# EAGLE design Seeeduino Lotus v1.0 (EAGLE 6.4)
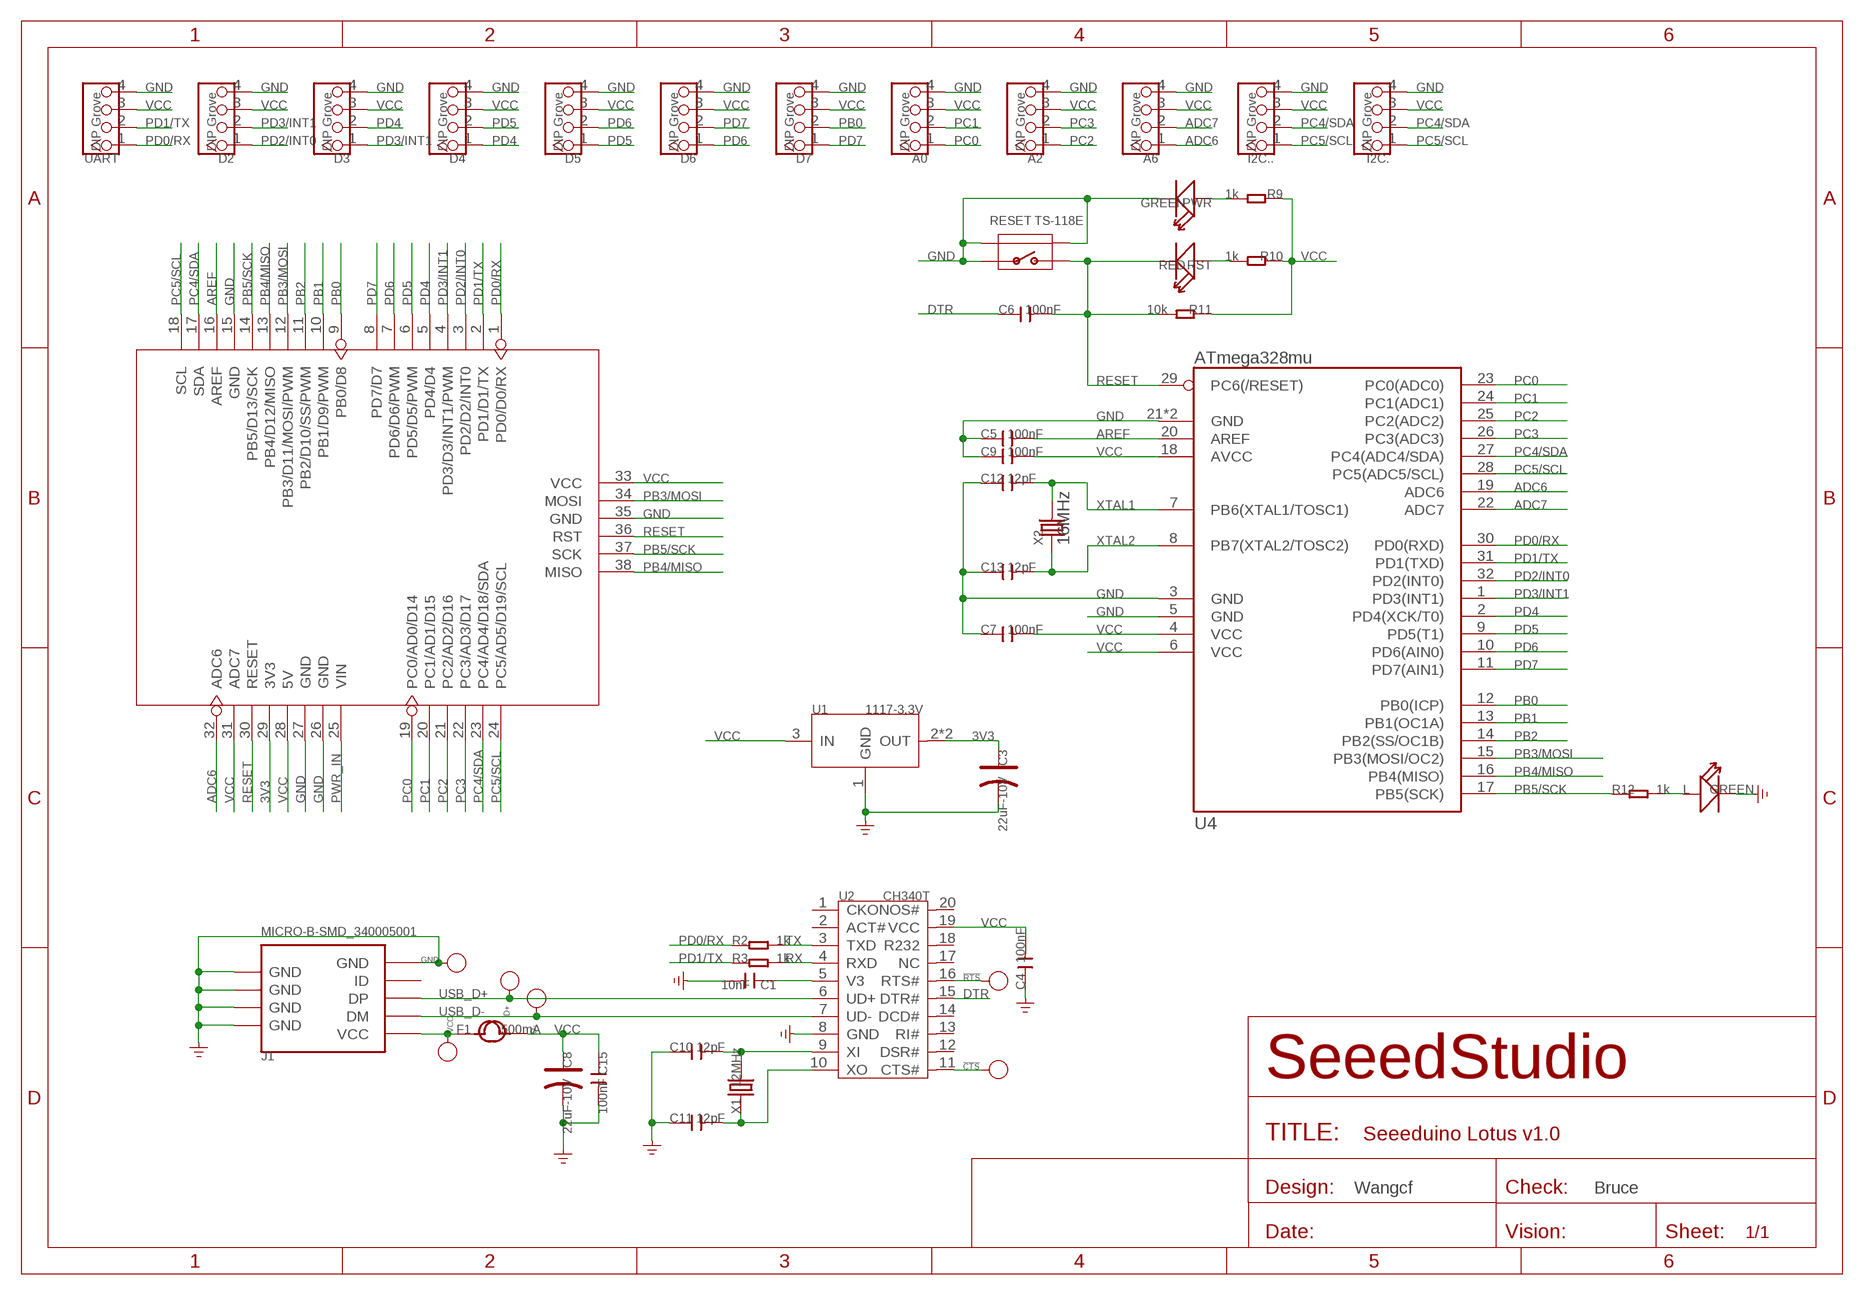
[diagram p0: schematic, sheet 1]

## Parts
!CTS  PAD-TEST-POINT'4545'  [TP_4545]
!RTS  PAD-TEST-POINT'4545'  [TP_4545]
A0  DIP Grove  TWIG-4P-2.0-2.0  [4P-2.0]
A2  DIP Grove  TWIG-4P-2.0-2.0  [4P-2.0]
A6  DIP Grove  TWIG-4P-2.0-2.0  [4P-2.0]
C1  10nF  C-0603  [C0603]
C3  22uF-10V  CAP-AVX-A  [AVX-A]
C4  100nF  C-0603  [C0603]
C5  100nF  C-0603  [C0603]
C6  100nF  C-0603  [C0603]
C7  100nF  C-0603  [C0603]
C8  22uF-10V  CAP-AVX-A  [AVX-A]
C9  100nF  C-0603  [C0603]
C10  12pF  C-0603  [C0603]
C11  12pF  C-0603  [C0603]
C12  12pF  C-0603  [C0603]
C13  12pF  C-0603  [C0603]
C15  100nF  C-0603  [C0603]
D2  DIP Grove  TWIG-4P-2.0-2.0  [4P-2.0]
D3  DIP Grove  TWIG-4P-2.0-2.0  [4P-2.0]
D4  DIP Grove  TWIG-4P-2.0-2.0  [4P-2.0]
D5  DIP Grove  TWIG-4P-2.0-2.0  [4P-2.0]
D6  DIP Grove  TWIG-4P-2.0-2.0  [4P-2.0]
D7  DIP Grove  TWIG-4P-2.0-2.0  [4P-2.0]
D+  PAD-TEST-POINT'4545'  [TP_4545]
D-  PAD-TEST-POINT'4545'  [TP_4545]
F1  500mA  FUSE'1206'  [F1206]
GND  PAD-TEST-POINT'4545'  [TP_4545]
I2C.  DIP Grove  TWIG-4P-2.0-2.0  [4P-2.0]
I2C..  DIP Grove  TWIG-4P-2.0-2.0  [4P-2.0]
J1  MICRO-B-SMD_340005001  USB-MINIUSB-5P-MICRO  [MICRO-USB]
L  GREEN  LED'0603'  [LED-0603]
PWR  GREEN  LED'0603'  [LED-0603]
R2  1k  R-0603  [R0603]
R3  1k  R-0603  [R0603]
R9  1k  R-0603  [R0603]
R10  1k  R-0603  [R0603]
R11  10k  R-0603  [R0603]
R12  1k  R-0603  [R0603]
RESET  TS-118E  BUTTON-4P-REINFORCE'TS-1188E'  [4P-SMD-7X3.5X3.5H]
RST  RED  LED'0603'  [LED-0603]
U1  1117-3.3V  LD1117'SOT89'  [SOT89]
U2  CH340T  [SSOP20]
U3  ARDUINO-38P  [ARDUINO-38P]
U4  ATmega328mu  ATMEGA8/168/328MLF  [MLF32X-W/HEAT]
UART  DIP Grove  TWIG-4P-2.0-2.0  [4P-2.0]
VCC  PAD-TEST-POINT'4545'  [TP_4545]
X1  12MHz  CRYSTAL'5032'  [2P-SMD-5X3.2]
X2  16MHz  CRYSTAL'5032'  [2P-SMD-5X3.2]

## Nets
3V3: C3.+ U1.2(OUT) U1.4(OUT) U3.29(3V3)
ADC6: A6.1 U3.32(ADC6) U4.19(ADC6)
ADC7: A6.2 U4.22(ADC7)
AREF: C5.2 U3.16(AREF) U4.20(AREF)
CTS: !CTS.T U2.11(CTS#)
DTR: C6.1 U2.15(DTR#)
GND: A0.4 A2.4 A6.4 C1.2 C3.- C4.1 C5.1 C7.1 C8.- C9.1 C10.1 C11.1 C12.1 C13.1 C15.2 D2.4 D3.4 D4.4 D5.4 D6.4 D7.4 GND.T I2C..4 I2C...4 J1.5(GND) J1.S1(GND) J1.S2(GND) J1.S3(GND) J1.S4(GND) J1.S5(GND) J1.S6(GND) L.- PWR.- RESET.1 RESET.S1 RESET.S2 U1.1(GND) U2.8(GND) U3.15(GND) U3.26(GND) U3.27(GND) U3.35(GND) U4.3(GND) U4.5(GND) U4.21(GND) U4.HEAT(GND) UART.4
N$2: R10.2 RST.+
N$3: PWR.+ R9.2
N$4: C10.2 U2.9(XI) X1.2
N$5: C11.2 U2.10(XO) X1.1
N$11: !RTS.T U2.16(RTS#)
N$12 [usbvcc]: F1.1 J1.1(VCC) VCC.T
N$13: L.+ R12.2
PB0: D7.2 U3.9(PB0/D8) U4.12(PB0(ICP))
PB1: U3.10(PB1/D9/PWM) U4.13(PB1(OC1A))
PB2: U3.11(PB2/D10/SS/PWM) U4.14(PB2(SS/OC1B))
PB3/MOSI: U3.12(PB3/D11/MOSI/PWM) U3.34(MOSI) U4.15(PB3(MOSI/OC2))
PB4/MISO: U3.13(PB4/D12/MISO) U3.38(MISO) U4.16(PB4(MISO))
PB5/SCK: R12.1 U3.14(PB5/D13/SCK) U3.37(SCK) U4.17(PB5(SCK))
PC0: A0.1 U3.19(PC0/AD0/D14) U4.23(PC0(ADC0))
PC1: A0.2 U3.20(PC1/AD1/D15) U4.24(PC1(ADC1))
PC2: A2.1 U3.21(PC2/AD2/D16) U4.25(PC2(ADC2))
PC3: A2.2 U3.22(PC3/AD3/D17) U4.26(PC3(ADC3))
PC4/SDA: I2C..2 I2C...2 U3.17(SDA) U3.23(PC4/AD4/D18/SDA) U4.27(PC4(ADC4/SDA))
PC5/SCL: I2C..1 I2C...1 U3.18(SCL) U3.24(PC5/AD5/D19/SCL) U4.28(PC5(ADC5/SCL))
PD0/RX: R2.1 U3.1(PD0/D0/RX) U4.30(PD0(RXD)) UART.1
PD1/TX: R3.1 U3.2(PD1/D1/TX) U4.31(PD1(TXD)) UART.2
PD2/INT0: D2.1 U3.3(PD2/D2/INT0) U4.32(PD2(INT0))
PD3/INT1: D2.2 D3.1 U3.4(PD3/D3/INT1/PWM) U4.1(PD3(INT1))
PD4: D3.2 D4.1 U3.5(PD4/D4) U4.2(PD4(XCK/T0))
PD5: D4.2 D5.1 U3.6(PD5/D5/PWM) U4.9(PD5(T1))
PD6: D5.2 D6.1 U3.7(PD6/D6/PWM) U4.10(PD6(AIN0))
PD7: D6.2 D7.1 U3.8(PD7/D7) U4.11(PD7(AIN1))
PWR_IN: U3.25(VIN)
RESET: C6.2 R11.2 RESET.2 RST.- U3.30(RESET) U3.36(RST) U4.29(PC6(/RESET))
RX: R3.2 U2.4(RXD)
TX: R2.2 U2.3(TXD)
USB_D+: D+.T J1.3(DP) U2.6(UD+)
USB_D-: D-.T J1.2(DM) U2.7(UD-)
V3: C1.1 U2.5(V3)
VCC: A0.3 A2.3 A6.3 C4.2 C7.2 C8.+ C9.2 C15.1 D2.3 D3.3 D4.3 D5.3 D6.3 D7.3 F1.2 I2C..3 I2C...3 R9.1 R10.1 R11.1 U1.3(IN) U2.19(VCC) U3.28(5V) U3.31(ADC7) U3.33(VCC) U4.4(VCC) U4.6(VCC) U4.18(AVCC) UART.3
XTAL1: C12.2 U4.7(PB6(XTAL1/TOSC1)) X2.2
XTAL2: C13.2 U4.8(PB7(XTAL2/TOSC2)) X2.1
Unconnected: J1.4(ID) U2.1(CKO) U2.2(ACT#) U2.12(DSR#) U2.13(RI#) U2.14(DCD#) U2.17(NC) U2.18(R232) U2.20(NOS#)

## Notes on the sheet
- Wangcf | Bruce

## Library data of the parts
!CTS !RTS D+ D- GND VCC = Discrete:PAD-TEST-POINT; PARTNO: DNP
A0 A2 A6 = Connector :TWIG-4P-2.0
C1 C4-C7 C9-C13 C15 = Discrete:C*: Ceramic Capacitors
C3 C8 = Discrete:CAP*: Electrolytic Capacitors,Tantalum Capacitors and Super Capacitors
D2-D7 I2C. I2C.. UART = Connector:TWIG-4P-2.0
F1 = Discrete:FUSE
J1 = Connector :USB-MINIUSB-5P
L PWR RST = Discrete:LED*
R2 R3 R9-R12 = Discrete:R*
RESET = Discrete:BUTTON-4P-REINFORCE: TS-1188E http://www.best-dz.com/?thread-374-2.html
U1 = IC:LD1117: Low Drop Fixed And Adjustable Positive Voltage Regulators http://www.datasheetcatalog.org/datasheet/SGSThomsonMicroelectronics/mXuqtqv.pdf
U2 = template:CH340T
U3 = moudle:ARDUINO-38P
U4 = IC:ATMEGA8/168/328: MICROCONTROLLER
X1 X2 = Discrete:CRYSTAL*: CRYSTAL

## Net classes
0 default: width 0.152 mm, drill 0.305 mm, clearance 0.152 mm
3 usbvcc: width 0.203 mm, drill 0.305 mm, clearance 0.203 mm

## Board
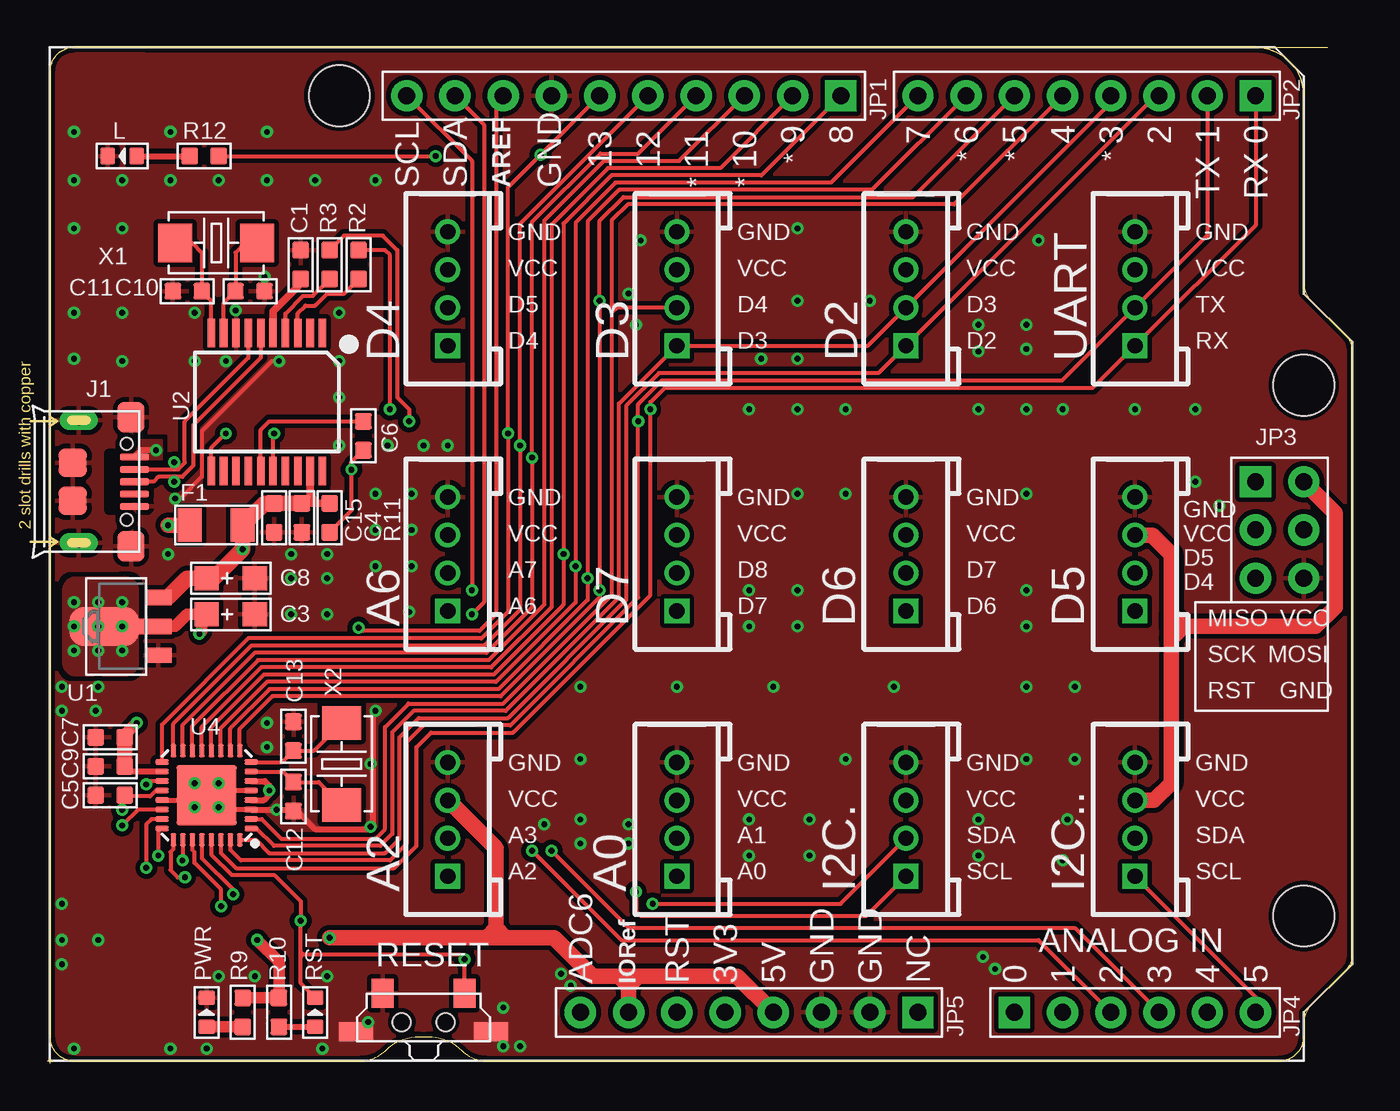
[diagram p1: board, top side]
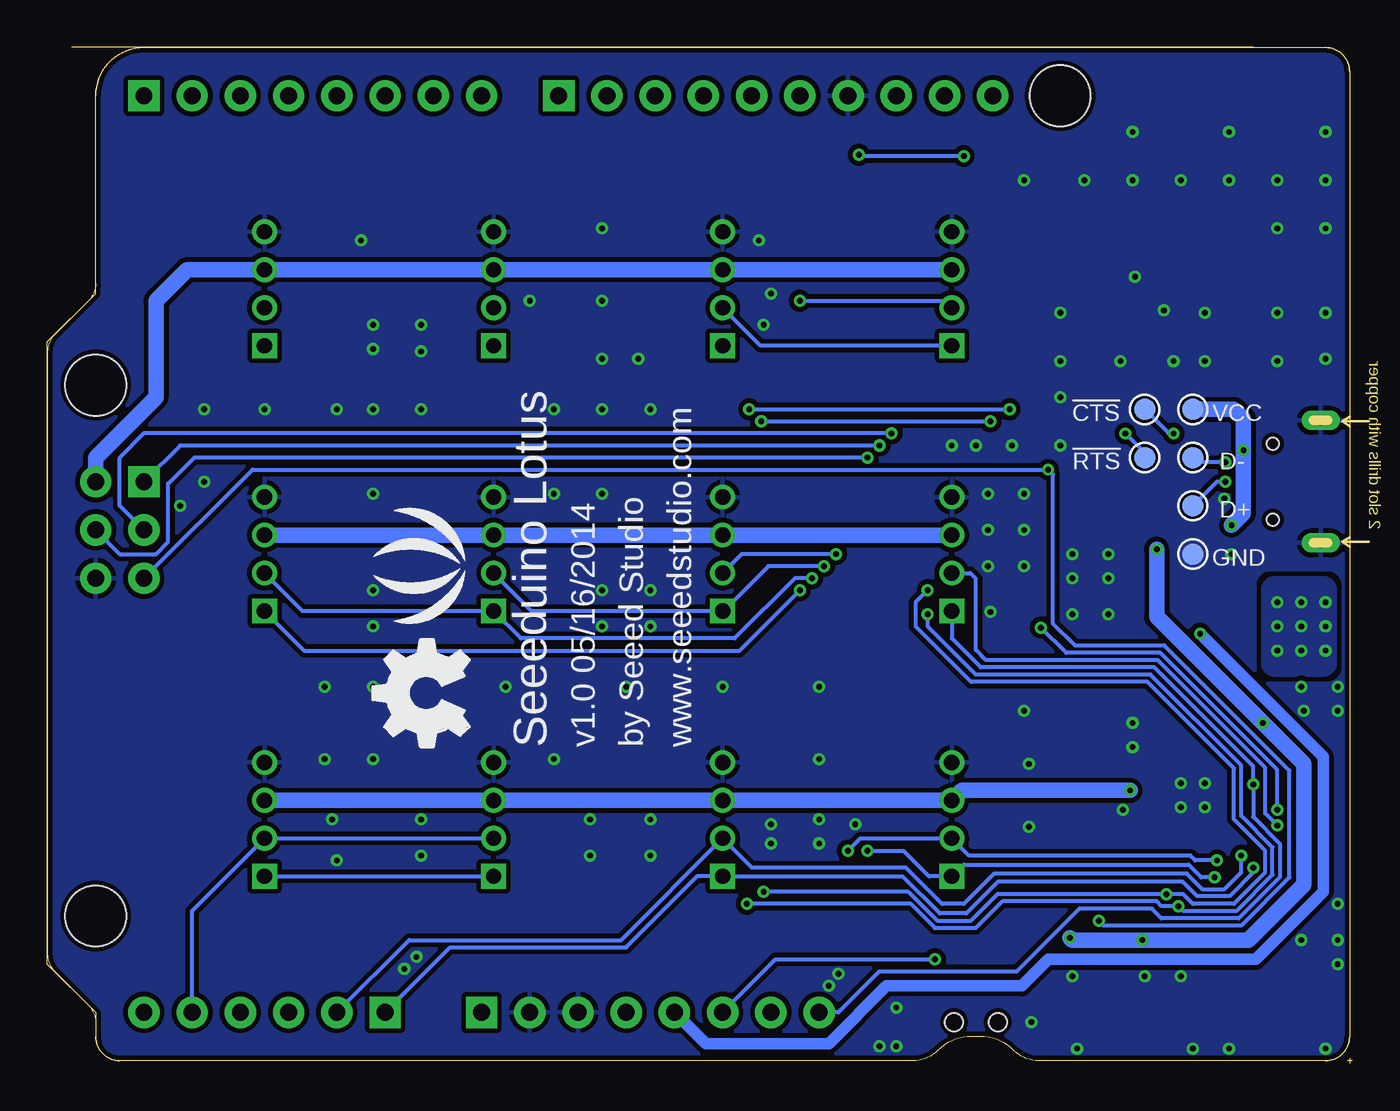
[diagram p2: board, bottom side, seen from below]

Size 68.71 x 53.47 mm. Coordinates in mm from the lower left corner, seen from the top.
Outline: 54 segments
Copper layers (1*16): Top 0.035mm / dielectric 1.5mm / Bottom 0.035mm
Design rules "SeeedStudio_rule_no_angle_090911 *": minimum track width 6mil, minimum drill 12mil, track to track 6mil, track to pad 6mil, pad to pad 6mil, via to via 6mil, smd to smd 0mil, copper to edge 10mil, drill to drill 10mil, minimum pad ring 10mil, minimum via ring 6mil, stop-mask expansion 2mil, vias tented up to drill 100mil, thermal gap 10mil

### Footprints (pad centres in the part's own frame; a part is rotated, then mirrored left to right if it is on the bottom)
TP_4545 = smd 1.143 x 1.143: T 0,0
4P-2.0 = drill 0.8 pad 1.27 square: 1 -3,0 | drill 0.8 pad 1.27: 2 -1,0; 3 1,0; 4 3,0
C0603 = smd 0.889 x 0.889: 1 -0.762,0; 2 0.762,0
AVX-A = smd 1.27 x 1.27: + -1.27,0; - 1.27,0
F1206 = smd 1.27 x 1.778: 1 -1.397,0; 2 1.397,0
MICRO-USB = smd 0.381 x 1.524: 1 -1.3,-0.25; 2 -0.65,-0.25; 3 0,-0.25; 4 0.65,-0.25; 5 1.3,-0.25 | smd 1.6 x 1.397: S1 -3.4,-0.427; S6 3.4,-0.427 | drill 0.508 pad 1.016 long: S2 -3.226,-3.175; S5 3.226,-3.175 | smd 1.5 x 1.5: S3 -1,-3.5; S4 1,-3.5 | hole 0.635: -2,-0.65; 2,-0.65
LED-0603 = smd 0.762 x 0.889: + -0.762,0; - 0.762,0
R0603 = smd 0.889 x 0.889: 1 -0.762,0; 2 0.762,0
4P-SMD-7X3.5X3.5H = smd 1.143 x 1.524: 1 -2.159,1.524; 2 2.159,1.524 | smd 1.778 x 1.016: S1 -3.556,-0.508; S2 3.556,-0.508 | hole 0.95: -1.15,0; 1.15,0
SOT89 = smd 0.8 x 1.4: 1 -1.524,-1.905; 3 1.524,-1.905 | smd 0.8 x 1.9: 2 0,-1.651 | smd 2.032 x 3.65: 4 0,0.94
SSOP20 = smd 0.4 x 1.5: 1 -2.925,-3.625; 2 -2.275,-3.625; 3 -1.625,-3.625; 4 -0.975,-3.625; 5 -0.325,-3.625; 6 0.325,-3.625; 7 0.975,-3.625; 8 1.625,-3.625; 9 2.275,-3.625; 10 2.925,-3.625; 11 2.925,3.625; 12 2.275,3.625; 13 1.625,3.625; 14 0.975,3.625; 15 0.325,3.625; 16 -0.325,3.625; 17 -0.975,3.625; 18 -1.625,3.625; 19 -2.275,3.625; 20 -2.925,3.625
ARDUINO-38P = drill 0.889 pad 1.651 square: 1 63.5,50.8; 9 41.656,50.8; 19 50.8,2.54; 25 45.72,2.54; 38 63.5,30.48 | drill 0.889 pad 1.651: 2 60.96,50.8; 3 58.42,50.8; 4 55.88,50.8; 5 53.34,50.8; 6 50.8,50.8; 7 48.26,50.8; 8 45.72,50.8; 10 39.116,50.8; 11 36.576,50.8; 12 34.036,50.8; 13 31.496,50.8; 14 28.956,50.8; 15 26.416,50.8; 16 23.876,50.8; 17 21.336,50.8; 18 18.796,50.8; 20 53.34,2.54; 21 55.88,2.54; 22 58.42,2.54; 23 60.96,2.54; 24 63.5,2.54; 26 43.18,2.54; 27 40.64,2.54; 28 38.1,2.54; 29 35.56,2.54; 30 33.02,2.54; 31 30.48,2.54; 32 27.94,2.54; 33 66.04,30.48; 34 66.04,27.94; 35 66.04,25.4; 36 63.5,25.4; 37 63.5,27.94 | hole 3.2: 15.24,50.8; 66.04,35.56; 66.04,7.62
MLF32X-W/HEAT = smd 0.7 x 0.3: 1 -2.35,1.75; 2 -2.35,1.25; 3 -2.35,0.75; 4 -2.35,0.25; 5 -2.35,-0.25; 6 -2.35,-0.75; 7 -2.35,-1.25; 8 -2.35,-1.75; 17 2.35,-1.75; 18 2.35,-1.25; 19 2.35,-0.75; 20 2.35,-0.25; 21 2.35,0.25; 22 2.35,0.75; 23 2.35,1.25; 24 2.35,1.75 | smd 0.3 x 0.7: 9 -1.75,-2.35; 10 -1.25,-2.35; 11 -0.75,-2.35; 12 -0.25,-2.35; 13 0.25,-2.35; 14 0.75,-2.35; 15 1.25,-2.35; 16 1.75,-2.35; 25 1.75,2.35; 26 1.25,2.35; 27 0.75,2.35; 28 0.25,2.35; 29 -0.25,2.35; 30 -0.75,2.35; 31 -1.25,2.35; 32 -1.75,2.35 | smd 3.175 x 3.175: HEAT 0,0
2P-SMD-5X3.2 = smd 1.778 x 2.032: 1 -2.159,0; 2 2.159,0

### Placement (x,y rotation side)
!CTS  10.92,34.42 0 bottom
!RTS  10.92,31.88 0 bottom
A0  33.15,12.83 90 top
A2  21.08,12.83 90 top
A6  21.08,26.8 90 top
C1  13.34,42.04 90 top
C3  9.65,23.62 0 top
C4  13.4,28.7 90 top
C5  3.3,14.1 0 top
C6  16.64,33.02 270 top
C7  3.3,17.14 0 top
C8  9.65,25.53 0 top
C9  3.3,15.62 0 top
C10  10.67,40.64 180 top
C11  7.37,40.64 0 top
C12  12.95,14.03 90 top
C13  12.95,17.21 270 top
C15  11.94,28.7 270 top
D2  45.21,40.77 90 top
D3  33.15,40.77 90 top
D4  21.08,40.77 90 top
D5  57.28,26.8 90 top
D6  45.21,26.8 90 top
D7  33.15,26.8 90 top
D+  8.38,29.34 0 bottom
D-  8.38,31.88 0 bottom
F1  8.89,28.32 0 top
GND  8.38,26.8 0 bottom
I2C.  45.21,12.83 90 top
I2C..  57.28,12.83 90 top
J1  4.83,30.61 270 top
L  3.94,47.75 180 top
PWR  8.38,2.67 90 top
R2  16.38,42.04 270 top
R3  14.86,42.04 270 top
R9  10.29,2.67 270 top
R10  12.19,2.67 270 top
R11  14.86,28.7 270 top
R12  8.26,47.75 180 top
RESET  19.81,2.16 0 top
RST  14.1,2.67 90 top
U1  3.94,22.99 90 top
U2  11.56,34.8 180 top
U3  0.13,0.13 0 top
U4  8.38,14.1 180 top
U$2  [OSHW_FILLX200_NOTEXT]  46.48,16.64 90 bottom
U$4  [LOGO_SILK]  48.39,26.16 90 bottom
U$12  [SEEED_MASK]  3.94,2.67 0 top
UART  57.28,40.77 90 top
VCC  8.38,34.42 0 bottom
X1  8.89,43.18 0 top
X2  15.49,15.75 270 top

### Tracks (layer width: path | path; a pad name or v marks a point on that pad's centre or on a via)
3V3  (via drill 0.3 pad 0.64)
  Top 0.61: v8,22.61 8.13,22.73 8.13,23.49 8.26,23.62 | v3.94,22.99 U1.4 | 8.38,23.49 8.51,23.62 | U1.2 6.73,22.99 7.37,23.62 C3.+
  Top 0.813: 8.26,23.62 C3.+ 8.38,23.49
  Bottom 0.61: U3.29 34.04,1.02 27.56,1.02 24.51,4.06 17.4,4.06 16,5.46 5.08,5.46 1.52,9.02 1.52,16.13 v8,22.61
  other vias: 3.94,24.26 2.67,24.26 1.4,24.26 2.67,22.99 1.4,22.99 1.4,21.72 2.67,21.72 3.94,21.72
  pour Top (isolate 0.254, no thermals): 4.06,20.45 1.52,20.45 arc-90 0.89,21.08 0.89,24.89 arc-90 1.52,25.53 4.06,25.53 arc-90 4.7,24.89 4.7,21.08 arc-90
  pour Bottom (isolate 0.254, no thermals): 4.06,20.45 1.52,20.45 arc-90 0.89,21.08 0.89,24.89 arc-90 1.52,25.53 4.06,25.53 arc-90 4.7,24.89 4.7,21.08 arc-90
ADC6  (via drill 0.3 pad 0.64)
  Top 0.203: U4.19 5.38,14.85 v5.21,14.67
  Bottom 0.203: U3.32 27.05,2.67 24.89,4.83 17.65,4.83 14.35,8.13 10.54,8.13 10.03,7.62 5.97,7.62 3.81,9.78 3.81,11.56 5.21,12.95 v5.21,14.67 5.21,15.63 10.41,20.83 19.56,20.83 21.08,22.35 A6.1
ADC7  (via drill 0.3 pad 0.64)
  Top 0.203: U4.22 4.77,13.35 v3.94,12.51
  Bottom 0.203: A6.2 20.1,25.8 19.81,25.51 19.81,21.75 19.27,21.21 10.24,21.21 4.57,15.54 4.57,13.15 v3.94,12.51
AREF  (via drill 0.3 pad 0.64)
  Top 0.203: U3.16 23.62,50.55 23.62,23.62 22.75,22.75 16.62,22.75 16.45,22.92 v16.38,22.92 | U4.20 5.71,14.35 5.4,14.03 4.13,14.03 C5.2 3.94,13.97 v3.94,13.34
  Bottom 0.203: v3.94,13.34 3.94,15.43 10.1,21.59 15.05,21.59 v16.38,22.92
CTS  (via drill 0.3 pad 0.61)
  Top 0.203: U2.11 8.63,32.38 v9.4,33.15
  Bottom 0.203: v9.4,33.15 9.65,33.15 !CTS.T
DTR
  Top 0.203: U2.15 11.23,33.33 11.68,33.78 C6.1
GND  (via drill 0.3 pad 0.64)
  Top 0.203: v12.19,36.96 11.81,36.96 8.13,33.27 8.13,30.86 6.98,29.72 v6.73,29.72
  Top 0.254: U4.21 6.86,13.85 v7.75,14.73 U4.HEAT | U4.3 9.13,13.35 v9.02,13.46 | U4.5 9.4,14.35 v9.02,14.73
  Top 0.305: U4.3 12.88,13.35 C12.1 13.15,13.27 14.1,12.32 16.89,12.32 17.14,12.57 17.14,18.54
  other vias: 14.48,0.76 16.89,2.16 24.89,0.89 36.96,24.89 39.5,24.89 39.5,22.99 36.96,22.99 51.56,24.89 51.56,22.99 49.02,12.83 40.13,10.92 53.72,12.83 49.02,10.92 40.13,12.83 53.47,10.67 26.16,12.57 30.61,12.57 27.05,4.7 27.56,4.06 24,0.89 1.4,43.94 3.94,43.94 1.4,49.02 17.27,28.07 60.45,30.61 61.72,29.34 37.59,37.08 39.5,37.08 30.99,38.86 30.61,40.51 31.24,43.31 49.28,5.59 49.91,4.95 1.4,39.5 3.94,39.5 19.81,32.51 21.08,32.51 30.61,11.56 36.96,10.92 36.96,12.83 49.02,37.47 49.02,38.86 7.75,13.46 11.56,17.91 0.76,19.81 2.67,19.81 0.76,18.54 0.76,6.48 0.76,8.38 2.67,6.48 1.4,0.76 6.48,0.76 8.38,0.76 14.73,4.57 12.83,25.53 12.83,23.62 14.73,23.62 2.54,18.54 17.27,18.54 17.02,15.75 12.07,13.34 17.02,12.45 3.94,46.48 1.4,46.48 6.48,46.48 9.02,46.48 11.56,46.48 14.1,46.48 17.27,46.48 6.48,49.02 11.56,49.02 1.4,37.08 9.91,39.62 11.43,41.4 15.37,32.51 15.37,35.05 17.91,32.51 9.4,36.96 15.37,36.96 28.07,11.56 28.07,12.83 28.07,16 28.07,19.81 33.15,19.81 38.23,19.81 44.58,19.81 51.56,19.81 54.1,19.81 54.1,16 51.56,16 42.04,16 36.96,34.42 39.5,34.42 42.04,34.42 43.31,40.13 39.5,40.13 39.5,43.94 52.2,43.31 51.56,38.86 51.56,37.59 49.02,34.42 51.56,34.42 53.47,34.42 60.45,34.42 57.28,34.42 17.27,29.97 19.18,29.97 19.18,28.07 17.27,26.16 19.05,23.75 19.18,26.16 51.56,29.97 39.5,29.97 42.04,29.97 7.75,39.5 7.75,36.96 15.37,39.5 9.02,4.57 10.92,4.57 0.76,5.21 14.73,25.53 14.73,26.8 12.83,26.8 6.35,26.8 11.56,16.64 3.94,36.96 24,2.92
  pour Bottom (isolate 0.254, rank 6): 0.13,0.13 68.71,0.13 68.71,53.47 0.13,53.47
  pour Top (isolate 0.254, rank 6): 0.13,0.13 68.71,0.13 68.71,53.47 0.13,53.47
N$2
  Top 0.305: R10.2 RST.+
N$3
  Top 0.61: PWR.+ R9.2
N$4
  Top 0.203: U2.9 9.28,40.02 C10.2 9.91,42.67 10.41,43.18 X1.2
N$5
  Top 0.203: U2.10 8.63,40.14 C11.2 8.13,42.67 7.62,43.18 X1.1
N$11  (via drill 0.3 pad 0.61)
  Top 0.203: U2.16 11.88,33.09 v11.94,33.15
  Bottom 0.203: !RTS.T 10.92,32.13 v11.94,33.15
N$12  (via drill 0.3 pad 0.64)
  Top 0.305: v5.71,32.26 4.93,32.26 J1.1
  Top 0.813: v6.35,28.32 F1.1
  Bottom 0.813: VCC.T 6.22,34.42 5.71,33.91 v5.71,32.26 5.71,28.96 v6.35,28.32
  pour Top (isolate 0.254, no thermals): 3.81,32.77 5.97,32.77 5.97,31.81 3.81,31.81
N$13
  Top 0.305: L.+ R12.2
PB0  (via drill 0.3 pad 0.64)
  Top 0.203: U3.9 37.59,46.74 29.72,46.74 27.18,44.2 v27.18,26.8 27.18,24.13 23.49,20.45 11.39,20.45 8.63,17.69 U4.12
  Bottom 0.203: v27.18,26.8 32.15,26.8 D7.2
PB1
  Top 0.203: U3.10 35.43,47.12 29.52,47.12 26.54,44.14 26.54,24 23.37,20.83 11.26,20.83 8.13,17.7 U4.13
PB2
  Top 0.203: U3.11 33.27,47.5 29.32,47.5 26.16,44.34 26.16,24.13 23.24,21.21 11.09,21.21 7.63,17.75 U4.14
PB3/MOSI  (via drill 0.3 pad 0.64)
  Top 0.203: U4.15 7.13,17.82 10.9,21.59 23.11,21.59 25.53,24 v25.53,31.88 25.53,44.28 29.12,47.88 31.11,47.88 U3.12
  Bottom 0.203: U3.34 64.9,26.8 62.99,26.8 62.36,27.43 62.36,30.5 60.98,31.88 v25.53,31.88
PB4/MISO  (via drill 0.3 pad 0.64)
  Top 0.203: U4.16 6.63,17.87 10.73,21.97 22.99,21.97 24.89,23.88 v24.89,32.51 24.89,44.2 U3.13
  Bottom 0.203: v24.89,32.51 61.72,32.51 U3.38
PB5/SCK  (via drill 0.3 pad 0.64)
  Top 0.203: U4.17 6.03,17.82 10.56,22.35 22.86,22.35 24.26,23.75 v24.26,33.15 24.26,46.1 v25.97,47.82 U3.14 | R12.1 v20.45,47.75
  Bottom 0.203: U3.37 64.9,29.34 64.9,31.88 63.63,33.15 v24.26,33.15 | v20.45,47.75 25.91,47.75 v25.97,47.82
PC0  (via drill 0.3 pad 0.64)
  Top 0.203: U4.23 5.48,12.85 5.21,12.57 v5.21,10.29
  Bottom 0.203: U3.19 47.5,6.1 38.23,6.1 34.5,9.83 A0.1 23.67,9.83 21.72,7.87 20.32,7.87 18.66,9.54 8.9,9.54 8.16,8.79 6.45,8.79 5.21,10.03 v5.21,10.29
PC1  (via drill 0.3 pad 0.64)
  Top 0.203: U4.24 5.87,12.35 5.84,12.32 v5.84,10.92
  Bottom 0.203: U3.20 49.66,6.48 38.5,6.48 A0.2 31.61,10.29 23.49,10.29 21.59,8.38 20.45,8.38 18.86,9.97 8.7,9.97 7.89,9.16 6.72,9.16 5.84,10.03 v5.84,10.92
PC2  (via drill 0.3 pad 0.64)
  Top 0.203: U4.25 6.63,11.27 6.48,11.11 6.48,10.16 6.86,9.78 v7.24,9.78 | v25.53,11.18 30.23,6.48 52.2,6.48 U3.21
  Bottom 0.203: v25.53,11.18 23.62,11.18 22.27,9.83 A2.1 21.03,9.83 20.42,10.44 8.6,10.44 7.94,9.78 v7.24,9.78
PC3  (via drill 0.3 pad 0.64)
  Top 0.203: U3.22 54.1,7.11 30.61,7.11 v26.54,11.18 | U4.26 7.13,10.69 v7.11,10.67
  Bottom 0.203: v26.54,11.18 25.91,11.81 21.1,11.81 A2.2 20.18,10.92 8.51,10.92 8.26,10.67 v7.11,10.67
PC4/SDA  (via drill 0.3 pad 0.64)
  Top 0.203: v31.88,8.38 41.77,8.38 I2C..2 | U3.17 22.99,49.4 22.99,24.26 v22.35,23.62 | U4.27 7.63,11.23 7.75,11.11 7.75,10.54 9.14,9.14 v9.14,8.26
  Bottom 0.203: I2C..2 I2C...2 61.09,8.02 U3.23 | v31.88,8.38 23.24,8.38 21.97,7.11 19.81,7.11 18.41,8.51 10.29,8.51 10.03,8.26 v9.14,8.26 8.89,8 6.1,8 4.19,9.91 4.19,11.37 5.84,13.02 5.84,15.67 10.62,20.45 19.81,20.45 22.35,22.99 v22.35,23.62
PC5/SCL  (via drill 0.3 pad 0.64)
  Top 0.203: U3.24 63.63,3.48 I2C...1 | I2C..1 43.13,7.75 31.24,7.75 30.99,8 v30.99,9.02 | U3.18 22.35,47.5 v22.35,24.89 | U4.28 8.13,10.79 9.78,9.14 v9.78,8.89
  Bottom 0.203: I2C...1 I2C..1 | v30.99,9.02 23.37,9.02 21.84,7.49 20.07,7.49 18.67,8.89 v9.78,8.89 8.89,8.89 8.38,8.38 6.22,8.38 4.57,10.03 4.57,11.18 6.22,12.83 6.22,15.52 10.77,20.07 20.07,20.07 22.99,22.99 22.99,24.26 v22.35,24.89
PD0/RX  (via drill 0.3 pad 0.64)
  Top 0.203: U3.1 63.63,44.12 UART.1 55.07,35.56 32.51,35.56 31.75,34.8 v31.75,34.42 31.75,24.64 24.51,17.4 20.19,17.4 19.43,16.64 19.43,11.43 18.26,10.26 9.94,10.26 9.13,11.07 U4.30 | v18.03,34.42 18.03,42.55 17.78,42.8 R2.1
  Bottom 0.203: v31.75,34.42 v18.03,34.42
PD1/TX  (via drill 0.3 pad 0.64)
  Top 0.203: U3.2 61.09,43.58 UART.2 53.45,35.94 32.37,35.94 31.11,34.68 v31.11,33.78 31.11,24.51 24.38,17.78 19.81,17.78 18.92,16.89 18.92,11.56 18.03,10.67 10.19,10.67 9.63,11.22 U4.31 | v19.05,33.78 19.05,34.42 18.41,35.05 18.41,42.8 17.65,43.56 15.62,43.56 R3.1
  Bottom 0.203: v31.11,33.78 v19.05,33.78
PD2/INT0
  Top 0.203: U3.3 58.37,50.93 D2.1 43.77,36.32 32.21,36.32 30.48,34.6 30.48,24.38 24.26,18.16 19.56,18.16 18.54,17.14 18.54,11.81 17.78,11.05 11.68,11.05 10.99,11.75 U4.32 10.13,11.59
PD3/INT1
  Top 0.203: U3.4 56.01,50.56 D2.2 43.21,37.77 D3.1 30.1,34.72 30.1,24.51 24.13,18.54 19.28,18.54 18.16,17.42 18.16,12.07 17.53,11.43 11.94,11.43 11.02,12.35 U4.1
PD4
  Top 0.203: U3.5 47.75,45.21 30.57,45.21 29.72,44.36 29.72,40.01 | 29.72,40.01 29.72,39.75 | D3.2 29.99,39.77 | 29.96,39.77 29.73,39.77 29.72,39.75 | 29.72,39.5 29.72,24.64 24,18.92 19.01,18.92 17.78,17.69 17.78,12.32 17.27,11.81 12.32,11.81 11.28,12.85 U4.2 | 29.99,39.77 29.96,39.77 | 29.96,39.77 29.72,40.01 | 29.99,39.77 29.72,39.5 | 29.72,39.5 29.72,39.75
  Bottom 0.203: D4.1 31.15,37.77 D3.2
PD5  (via drill 0.3 pad 0.64)
  Top 0.203: U3.6 45.59,45.59 30.33,45.59 29.08,44.34 v29.08,40.13 v29.08,24.89 29.08,24.51 23.88,19.3 11.84,19.3 10.13,17.6 U4.9 10.1,16.48
  Bottom 0.203: D5.1 55.2,21.72 32.26,21.72 v29.08,24.89 | v29.08,40.13 21.45,40.13 D4.2
PD6  (via drill 0.3 pad 0.64)
  Top 0.203: U3.7 43.43,45.97 30.1,45.97 28.45,44.32 v28.45,25.53 28.45,24.38 23.75,19.68 11.7,19.68 9.63,17.62 U4.10
  Bottom 0.203: D5.2 55.28,23.8 D6.1 43.77,22.35 32.51,22.35 29.34,25.53 v28.45,25.53
PD7  (via drill 0.3 pad 0.64)
  Top 0.203: U3.8 41.28,46.36 29.91,46.36 27.81,44.25 v27.81,26.16 27.81,24.26 23.62,20.07 11.57,20.07 9.13,17.63 U4.11
  Bottom 0.203: D6.2 43.21,23.8 D7.1 33.1,23.8 30.73,26.16 v27.81,26.16
RESET  (via drill 0.3 pad 0.61, 0.3 pad 0.64)
  Top 0.203: U4.29 8.63,10.98 9.7,9.91 11.94,9.91 13.34,8.51 v13.34,7.49 13.34,5.84 | RST.- 13.34,4.19 13.34,5.59 | 13.34,5.59 13.34,5.84 | 13.46,5.71 13.34,5.84 | 13.46,5.71 21.72,5.71 v21.97,5.46 RESET.2 | 13.46,5.71 13.34,5.59 | R11.2 16,29.08 v16,31.24 16,31.62 C6.2
  Bottom 0.203: U3.30 30.35,5.46 v21.97,5.46 | U3.36 57.91,31.24 v16,31.24 15.75,30.99 15.75,23.14 14.58,21.97 9.88,21.97 3.3,15.4 3.3,9.76 3.32,9.76 5.84,7.24 13.08,7.24 v13.34,7.49
RX
  Top 0.203: U2.4 12.53,39.46 13.46,40.39 13.97,40.39 R3.2
TX
  Top 0.203: U2.3 13.18,39.47 13.59,39.88 14.1,39.88 14.73,40.51 15.62,40.51 R2.2
USB_D+  (via drill 0.3 pad 0.64)
  Top 0.203: U2.6 11.23,37.14 7.68,33.59 7.68,31.45 7.1,30.86 6.73,30.86 | 6.73,30.86 5.84,30.86 5.59,30.61 J1.3 | v6.67,30.61 6.67,30.8 6.73,30.86
  Bottom 0.203: 8.38,29.46 D+.T 7.11,30.61 v6.67,30.61
USB_D-  (via drill 0.3 pad 0.64)
  Top 0.203: J1.2 6.6,31.26 | 6.6,31.26 6.89,31.26 7.24,31.61 7.24,33.78 10.58,37.12 U2.7 | v6.67,31.62 6.67,31.32 6.6,31.26
  Bottom 0.203: v6.67,31.62 8.13,31.62 D-.T
V3
  Top 0.406: U2.5 11.88,39.57 13.21,40.89 13.21,41.15 C1.1
VCC  (via drill 0.3 pad 0.64)
  Top 0.305: U4.18 4.34,15.35 C9.2 | U4.6 11.44,14.85 11.68,14.61 v11.68,14.35 11.68,14.13 11.4,13.85 U4.4
  Top 0.406: 21,27.88 A6.3 | U2.19 13.83,29.86 | 13.83,29.86 13.83,29.83 13.46,29.46 | 13.46,29.46 C4.2 | 13.46,29.46 14.22,29.46 | 14.22,29.46 R11.1 | 13.83,29.86 14.22,29.46
  Top 0.61: 21.07,27.81 A6.3 | R9.1 R10.1 12.19,5.33 v11.05,6.48 | C7.2 4.06,17.27 v4.7,17.91
  Top 0.813: D5.3 58.18,27.8 59.18,26.8 59.18,23.62 | 59.18,22.99 59.18,22.35 | 59.18,22.35 59.18,14.73 58.28,13.83 I2C...3 | U3.33 67.82,28.96 67.82,24 66.8,22.99 59.82,22.99 | 59.82,22.99 59.18,22.99 | 59.82,22.99 59.18,23.62 | 59.82,22.99 59.18,22.35 | 59.18,22.99 59.18,23.62 | U3.28 36.32,4.57 31.11,4.57 | 31.11,4.57 30.1,4.57 | 30.1,4.57 28.7,4.57 26.67,6.6 24.13,6.6 | U3.31 30.61,4.06 | 30.61,4.06 31.11,4.57 | 30.61,4.06 30.1,4.57 | 24.13,6.6 23.11,6.6 | A2.3 21.1,13.83 23.62,11.3 23.62,7.11 | 23.62,7.11 23.11,6.6 | 23.62,7.11 24.13,6.6 | 23.11,6.6 v14.86,6.6 | C7.2 C9.2 | U1.3 6.35,24.51 7.37,25.53 C8.+ 8.76,25.53 v10.29,27.05 F1.2 | 10.29,28.45 F1.2 | F1.2 11.43,29.46 C15.1 C4.2
  Bottom 0.813: A6.3 D7.3 D6.3 D5.3 | D4.3 D3.3 D2.3 UART.3 61.36,41.77 62.99,40.13 62.99,35.05 66.17,31.88 U3.33 | I2C...3 I2C..3 A0.3 A2.3 20.56,14.35 v11.68,14.35 | v14.86,6.6 14.73,6.48 v11.05,6.48 5.46,6.48 2.54,9.4 2.54,15.75 v4.7,17.91 10.29,23.49 v10.29,27.05
XTAL1
  Top 0.203: U4.7 12.4,15.35 C12.2 14.29,14.79 X2.2
XTAL2
  Top 0.203: U4.8 12.35,15.85 C13.2 14.03,16.45 X2.1

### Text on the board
tPlace: 9 | 8 | 7 | 6 | 5 | 4 | 3 | 2 | 1 | 0 | 13 | 12 | 11 | 10 | * | * | * | * | SCL | SDA | AREF | GND | * | * | TX | RX | GND | GND | GND | GND | VCC | VCC | VCC | VCC | D5 | D4 | D3 | TX | D4 | D3 | D2 | RX | GND | GND | GND | GND | VCC | VCC | VCC | VCC | D5 | A7 | D8 | D7 | D4 | A6 | D7 | D6 | MISO | VCC | SCK | MOSI | RST | GND | GND | GND | GND | GND | VCC | VCC | VCC | VCC | A3 | A1 | SDA | SDA | A2 | A0 | SCL | SCL | ANALOG IN | ADC6 | IORef | RST | 3V3 | 5V | GND | GND | NC | 0 | 1 | 2 | 3 | 4 | 5
bPlace: www.seeedstudio.com | by Seeed Studio | v1.0 05/16/2014 | Seeeduino Lotus
bPlate: A0 | A2 | A4 | SPI | UART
